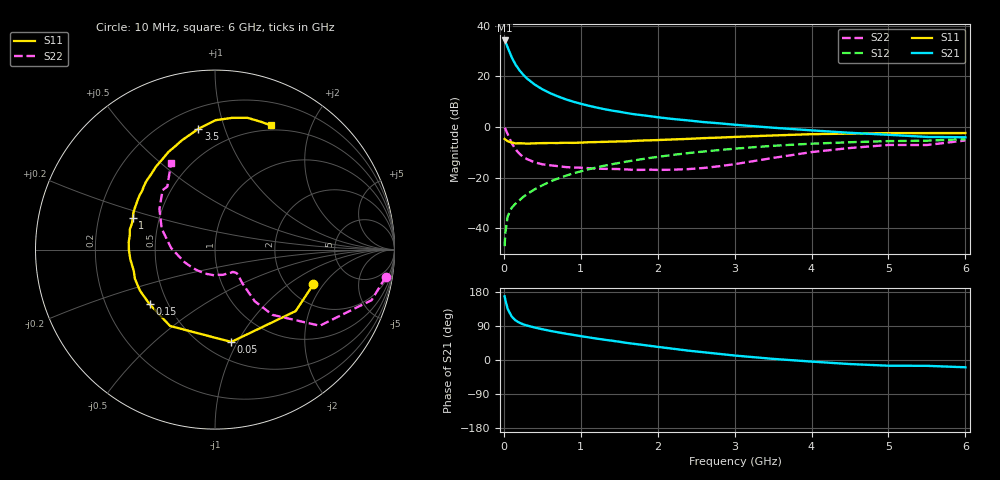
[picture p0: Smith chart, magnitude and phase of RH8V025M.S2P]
! SIEMENS Small Signal Semiconductors
! BFR106
! Si NPN RF Bipolar Junction Transistor in SOT23
! VCE = 8 V  IC = 25 mA
! Common Emitter S-Parameters:  August  1996
# GHz  S  MA  R  50
!  f  S11  S21  S12  S22
! GHz  MAG  ANG  MAG  ANG  MAG  ANG  MAG  ANG
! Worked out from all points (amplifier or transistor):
!   36 points, 10 MHz to 6 GHz, reference 50 ohm
!   highest |S21| = 34.2 dB at 10 MHz (marker M1)
!   |S21| within 3 dB of that: start of sweep to 53.14 MHz
!   unconditionally stable (mu >= 1): 350.1 MHz to 2.122 GHz
!   at 250 MHz: K = 0.91, MSG = 24.2 dB, |S12| = -27.7 dB
!   at 1.4 GHz: K = 1.06, MAG = 9.1 dB, |S12| = -14.8 dB
!   at 6 GHz: K = 0.98, MSG = 0.4 dB, |S12| = -4.8 dB
!   S11 on the Smith chart (normalised r, x): 10 MHz: 2.74, -1.60; 50 MHz: 0.67, -0.94; 150 MHz: 0.40, -0.31; 1 GHz: 0.35, +0.16; 3.5 GHz: 0.33, +0.82; 6 GHz: 0.44, +1.45
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0.01  0.5813 -19.4  51.38 167.9  0.0044 84.8  0.963 -9.1
0.02  0.5652 -37.3  48.5 158.2  0.0082 76.6  0.917 -17.9
0.05  0.5224 -80.0  37.36 135.0  0.0171 61.8  0.7215 -36.0
0.1  0.4937 -120.5  24.36 115.3  0.025 56.9  0.4848 -48.6
0.15  0.4747 -140.2  17.31 104.8  0.0304 56.3  0.3641 -52.4
0.2  0.4765 -151.3  13.42 98.8  0.0352 59.3  0.2992 -51.8
0.25  0.475 -160.1  10.85 94.2  0.0412 61.1  0.2552 -51.2
0.3  0.468 -165.1  9.108 91.0  0.0469 63.8  0.2323 -50.5
0.4  0.4751 -173.7  6.927 85.8  0.0585 65.7  0.2001 -48.5
0.5  0.4797 -179.6  5.568 81.2  0.0702 67.5  0.1832 -47.3
0.6  0.4825 175.0  4.669 77.0  0.0829 67.9  0.1749 -47.8
0.8  0.4879 166.8  3.547 69.6  0.1078 67.7  0.1615 -50.7
1  0.4905 158.9  2.881 63.0  0.1327 66.8  0.1568 -54.8
1.1  0.4992 155.6  2.637 59.8  0.1455 65.9  0.1536 -58.4
1.3  0.5073 149.7  2.261 53.7  0.1706 64.0  0.1487 -64.5
1.6  0.5223 140.9  1.881 45.1  0.2076 60.9  0.1448 -77.2
2.2  0.5674 125.4  1.438 29.7  0.281 53.5  0.1432 -108.4
2.8  0.6164 111.2  1.182 16.1  0.3499 45.0  0.1676 -147.4
3.5  0.6794 97.8  0.967 3.0  0.4249 34.8  0.2445 178.0
4.5  0.7401 82.6  0.767 -10.7  0.4995 19.4  0.3838 143.8
5.5  0.7568 70.1  0.636 -15.4  0.5363 8.7  0.4401 127.1
6  0.7589 65.9  0.626 -19.2  0.5763 1.2  0.5414 116.9
